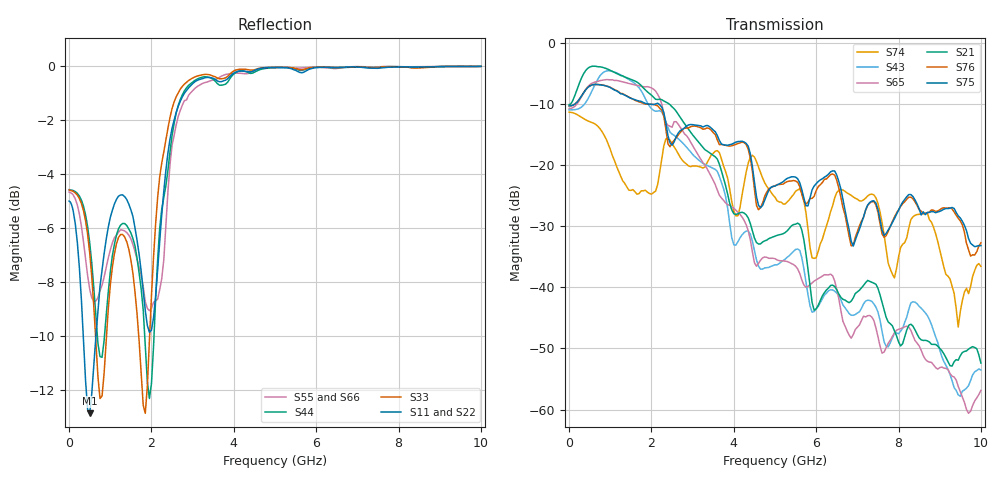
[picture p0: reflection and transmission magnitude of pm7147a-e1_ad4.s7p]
# GHz S DB R 50
! S-Parameters data
! Freq  dbS11  angS11  dbS12  angS12  dbS13  angS13  dbS14  angS14
!  dbS15  angS15  dbS16  angS16  dbS17  angS17  dbS21  angS21
!  dbS22  angS22  dbS23  angS23  dbS24  angS24  dbS25  angS25
!  dbS26  angS26  dbS27  angS27  dbS31  angS31  dbS32  angS32
!  dbS33  angS33  dbS34  angS34  dbS35  angS35  dbS36  angS36
!  dbS37  angS37  dbS41  angS41  dbS42  angS42  dbS43  angS43
!  dbS44  angS44  dbS45  angS45  dbS46  angS46  dbS47  angS47
!  dbS51  angS51  dbS52  angS52  dbS53  angS53  dbS54  angS54
!  dbS55  angS55  dbS56  angS56  dbS57  angS57  dbS61  angS61
!  dbS62  angS62  dbS63  angS63  dbS64  angS64  dbS65  angS65
!  dbS66  angS66  dbS67  angS67  dbS71  angS71  dbS72  angS72
!  dbS73  angS73  dbS74  angS74  dbS75  angS75  dbS76  angS76
!  dbS77  angS77
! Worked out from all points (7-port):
!   279 points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, 1 Hz to 10 GHz, reference 50 ohm
!   strongest paths, dB at 1 Hz, 7.943 MHz, 3.05 GHz, 6.55 GHz, 10 GHz:
!     S75: -10.3, -10.3, -13.5, -22.7, -33.2
!     S76: -10.3, -10.3, -13.6, -23.8, -32.7
!     S21: -10.1, -10.1, -15.5, -41.1, -52.4
!     S65: -10.8, -10.8, -17.4, -41.9, -56.9
!     S43: -11.0, -11.0, -18.6, -41.4, -53.5
!     S74: -11.4, -11.4, -20.2, -24.2, -36.6
!   lowest |S11| = -12.9 dB at 500 MHz (marker M1), VSWR 1.59, Z = 31.5 - j1.23 ohm
!   |S11| at or under -10 dB: 344 MHz to 651.9 MHz (307.9 MHz wide, 61.8 % of centre)
